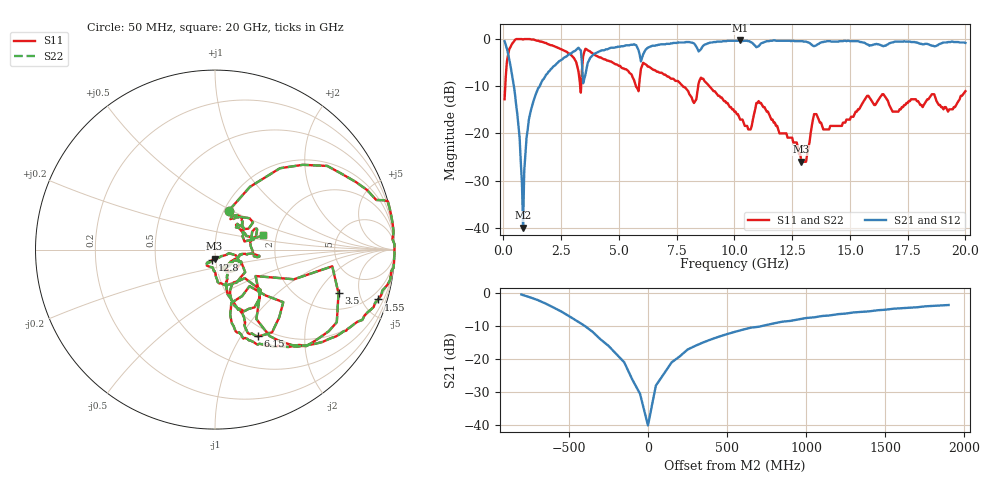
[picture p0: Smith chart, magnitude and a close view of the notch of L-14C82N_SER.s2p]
# MHZ S MA R 50
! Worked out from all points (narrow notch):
!   400 points, 50 MHz to 20 GHz, reference 50 ohm
!   highest |S21| = -0.26 dB at 10.25 GHz (marker M1); lowest = -40.0 dB at 850 MHz (marker M2)
!   notch at M2: 39.0 dB deep, 320 MHz wide at half that depth
!   lowest |S11| = -26.0 dB at 12.9 GHz (marker M3), VSWR 1.11, Z = 49.5 - j4.96 ohm
!   |S11| at or under -10 dB: 5.739 GHz to 5.87 GHz (130.7 MHz wide, 2.25 % of centre); 7.769 GHz to 8.431 GHz (662.7 MHz wide, 8.18 % of centre); 8.919 GHz to end of sweep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
!   |S22| runs from -26.0 to 0.0 dB; largest |S21 - S12| = 0
!   S11 on the Smith chart (normalised r, x): 50 MHz: 1.05, +0.48; 1.55 GHz: 1.14, -6.50; 3.5 GHz: 2.98, -3.11; 6.15 GHz: 0.87, -1.19; 12.8 GHz: 0.96, -0.11; 20 GHz: 1.70, +0.30
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50  0.23 70.5  0.95 -11.6  0.95 -11.6  0.23 70.5
250  0.78 36.7  0.61 -49.2  0.61 -49.2  0.78 36.7
600  1 13.3  0.16 -78.3  0.16 -78.3  1 13.3
850  0.99 3.4  0.01 57.5  0.01 57.5  0.99 3.4
900  1 1.8  0.04 68.9  0.04 68.9  1 1.8
1000  1 -1.4  0.09 80.0  0.09 80.0  1 -1.4
1550  0.95 -17.0  0.31 68.2  0.31 68.2  0.95 -17.0
3000  0.65 -53.1  0.73 36.0  0.73 36.0  0.65 -53.1
3400  0.47 -20.6  0.55 1.5  0.55 1.5  0.47 -20.6
3500  0.73 -19.5  0.38 21.6  0.38 21.6  0.73 -19.5
4250  0.63 -59.0  0.76 33.4  0.76 33.4  0.63 -59.0
5850  0.28 -46.7  0.76 2.7  0.76 2.7  0.28 -46.7
6150  0.54 -63.5  0.77 23.3  0.77 23.3  0.54 -63.5
6700  0.45 -68.2  0.87 16.0  0.87 16.0  0.45 -68.2
10050  0.17 -66.8  0.96 -3.5  0.96 -3.5  0.17 -66.8
10250  0.14 -62.3  0.97 -5.1  0.97 -5.1  0.14 -62.3
11050  0.22 -56.9  0.84 -3.6  0.84 -3.6  0.22 -56.9
12800  0.06 -105.9  0.95 -14.6  0.95 -14.6  0.06 -105.9
12900  0.05 -92.9  0.95 -15.3  0.95 -15.3  0.05 -92.9
13350  0.12 -15.3  0.87 -18.3  0.87 -18.3  0.12 -15.3
16700  0.2 14.8  0.9 -22.4  0.9 -22.4  0.2 14.8
20000  0.28 17.1  0.91 -41.5  0.91 -41.5  0.28 17.1
